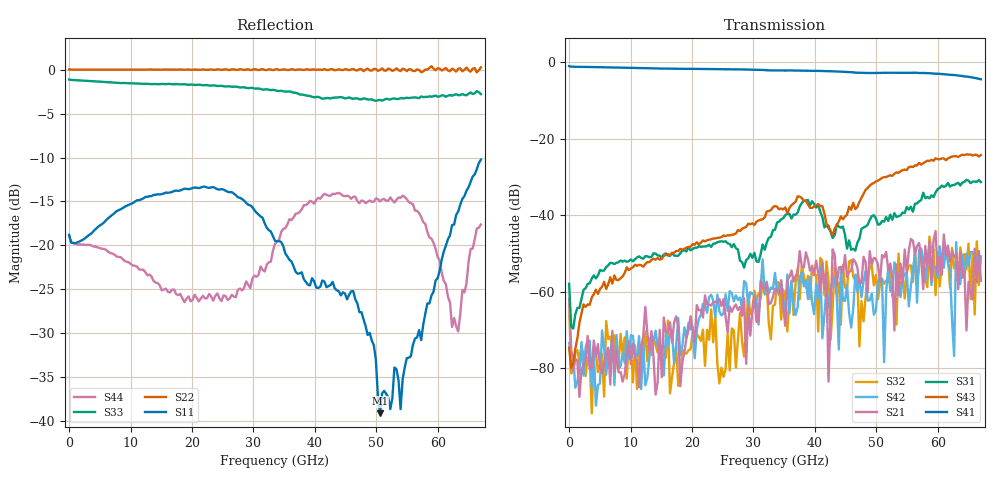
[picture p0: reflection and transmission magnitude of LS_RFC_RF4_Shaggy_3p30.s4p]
!Keysight Technologies,N5227A,US51270237,A.10.65.04
!Date: Tuesday, April 26, 2022 16:20:05
!Correction: S11(Full 4 Port(1,2,3,4))
!S12(Full 4 Port(1,2,3,4))
!S13(Full 4 Port(1,2,3,4))
!S14(Full 4 Port(1,2,3,4))
!S21(Full 4 Port(1,2,3,4))
!S22(Full 4 Port(1,2,3,4))
!S23(Full 4 Port(1,2,3,4))
!S24(Full 4 Port(1,2,3,4))
!S31(Full 4 Port(1,2,3,4))
!S32(Full 4 Port(1,2,3,4))
!S33(Full 4 Port(1,2,3,4))
!S34(Full 4 Port(1,2,3,4))
!S41(Full 4 Port(1,2,3,4))
!S42(Full 4 Port(1,2,3,4))
!S43(Full 4 Port(1,2,3,4))
!S44(Full 4 Port(1,2,3,4))
!S4P File: Measurements: <S11,S12,S13,S14>,
!<S21,S22,S23,S24>,
!<S31,S32,S33,S34>,
!<S41,S42,S43,S44>:
# Hz S  dB  R 50
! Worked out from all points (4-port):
!   201 points, 10 MHz to 67 GHz, reference 50 ohm
!   strongest paths, dB at 10 MHz, 16.76 GHz, 33.51 GHz, 50.25 GHz, 67 GHz:
!     S41: -1.1, -1.7, -2.2, -2.8, -4.5
!     S43: -74.5, -49.9, -37.6, -31.0, -24.3
!     S31: -57.9, -49.8, -43.8, -42.5, -31.4
!     S21: -61.8, -73.2, -59.2, -52.9, -57.1
!     S42: -73.3, -70.8, -55.1, -57.6, -50.8
!     S32: -63.2, -82.3, -63.3, -61.9, -51.3
!   lowest |S11| = -39.1 dB at 50.59 GHz (marker M1), VSWR 1.02, Z = 50 + j1.11 ohm
!   |S11| at or under -10 dB: start of sweep to end of sweep
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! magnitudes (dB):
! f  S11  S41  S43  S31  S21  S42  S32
! 10 MHz  -18.8  -1.1  -74.5  -57.9  -61.8  -73.3  -63.2
! 344.9 MHz  -19.7  -1.2  -79.9  -69.0  -74.7  -76.1  -81.3
! 50.59 GHz  -39.1  -2.9  -30.7  -42.4  -57.5  -56.2  -58.0
! 61.31 GHz  -20.0  -3.2  -25.6  -32.3  -50.5  -48.4  -49.9
! 62.65 GHz  -17.6  -3.4  -24.6  -32.1  -51.0  -76.7  -53.9
! 62.98 GHz  -16.5  -3.5  -24.6  -31.8  -50.0  -47.0  -52.4
! 67 GHz  -10.2  -4.5  -24.3  -31.4  -57.1  -50.8  -51.3
